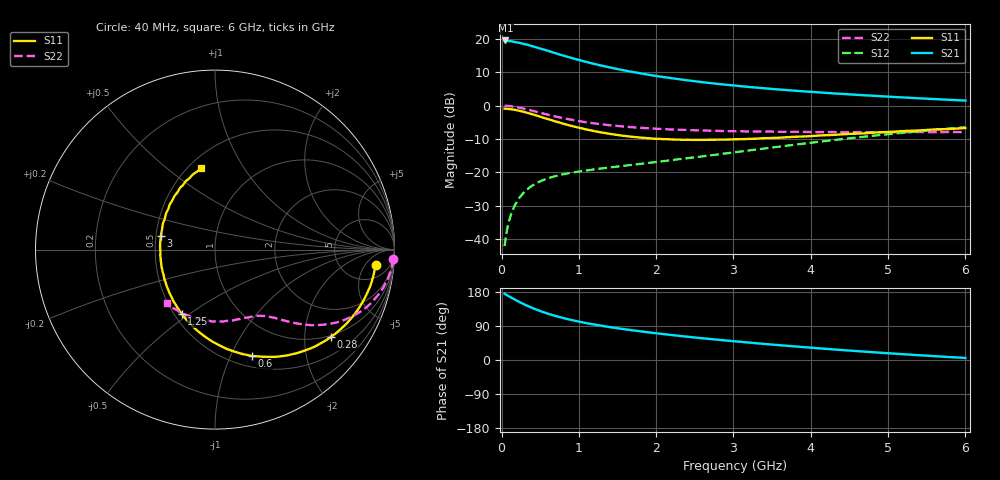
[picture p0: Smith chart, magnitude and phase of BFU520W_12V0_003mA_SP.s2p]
! Filename:  P:\Prog\Test\Noise\ATS_data\Testdata_Net\Run2\BFU520W_APM2013_06_A05_12p0V_003mA_SP_CM01_D.s2p
! Date/Time: Tue 26/Mar/2013 18:01:43
! BFU520W_APM2013_06_A05_12p0V_1to20mA_SP_CM01_Bias3_R.s2p
! MDIF S-parameter v. bias file
! BFU520W_APM2013_06_A05_12p0V_1to20mA_SP_CM01
! Date/time Thu Mar 21 16:35:01 2013
! VAR V_out= 12.0010
! VAR I_out= 2.9900
! VAR V_in= 0.8079
! VAR I_in= 0.0289
! Device data file deembeded for feedlines and parallel
! Original file: \Run2\BFU520W_APM2013_06_A05_12p0V_003mA_SP_CM01_R.s2p
! Feed-files: PR019V01_070313_Feed1.s2p, PR019V01_070313_Feed2.s2p
! Parallel-file: PR019V01_070313_Par.s2p
# MHz S MA R 50
!  Freq-MHz  S11-mag  S11-arg  S21-mag  S21-arg  S12-mag  S12-arg  S22-mag  S22-arg
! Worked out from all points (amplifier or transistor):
!   98 points, 40 MHz to 6 GHz, reference 50 ohm
!   highest |S21| = 19.5 dB at 50 MHz (marker M1)
!   |S21| within 3 dB of that: start of sweep to 586.1 MHz
!   unconditionally stable (mu >= 1): 2.183 GHz to 3.304 GHz
!   at 300 MHz: K = 0.23, MSG = 22.1 dB, |S12| = -25.8 dB
!   at 1.6 GHz: K = 0.89, MSG = 14.2 dB, |S12| = -18.0 dB
!   at 6 GHz: K = 0.84, MSG = 4.0 dB, |S12| = -6.5 dB
!   S11 on the Smith chart (normalised r, x): 40 MHz: 10, -9; 280 MHz: 0.95, -2.68; 600 MHz: 0.62, -1.20; 1.25 GHz: 0.55, -0.47; 3 GHz: 0.53, +0.09; 6 GHz: 0.58, +0.66
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40  0.8984 -5.5  9.429 174.9  0.0078 85.5  0.9941 -3.1
50  0.8972 -7.0  9.444 173.5  0.009657 85.0  0.9931 -4.0
140  0.8734 -19.3  9.125 163.0  0.0262 78.4  0.9683 -11.2
220  0.8394 -29.8  8.767 154.3  0.0395 72.9  0.9332 -16.9
280  0.8086 -37.1  8.392 148.2  0.04845 69.1  0.903 -20.8
340  0.7743 -44.4  8.11 142.6  0.05625 65.8  0.8682 -24.3
420  0.7269 -53.2  7.627 135.6  0.06544 62.1  0.8232 -28.3
500  0.6804 -61.5  7.148 129.3  0.07312 58.9  0.7794 -31.6
600  0.626 -71.0  6.613 122.3  0.08106 55.9  0.7284 -35.1
700  0.5767 -79.6  6.079 116.1  0.08762 53.6  0.6844 -38.0
800  0.534 -87.4  5.6 110.7  0.09322 52.1  0.6464 -40.2
900  0.4968 -94.8  5.186 105.8  0.09817 50.9  0.614 -42.1
1050  0.4511 -104.9  4.646 99.3  0.1045 50.1  0.572 -44.5
1250  0.4026 -117.3  4.071 91.8  0.1124 49.8  0.5312 -47.0
1600  0.3495 -136.7  3.338 80.9  0.1256 50.8  0.4824 -50.9
2050  0.3157 -157.9  2.718 69.3  0.1446 53.2  0.4458 -55.8
2500  0.3046 -176.8  2.311 59.4  0.1675 55.4  0.4255 -61.5
3000  0.3113 165.7  1.998 49.6  0.1983 57.0  0.4117 -68.9
3100  0.3137 162.3  1.945 47.8  0.2051 57.2  0.4111 -70.4
4100  0.3549 135.7  1.576 30.9  0.2858 55.8  0.399 -88.6
5200  0.4146 113.1  1.321 15.2  0.3919 48.7  0.3966 -112.2
6000  0.4596 99.5  1.186 5.5  0.4714 41.3  0.3993 -131.9
